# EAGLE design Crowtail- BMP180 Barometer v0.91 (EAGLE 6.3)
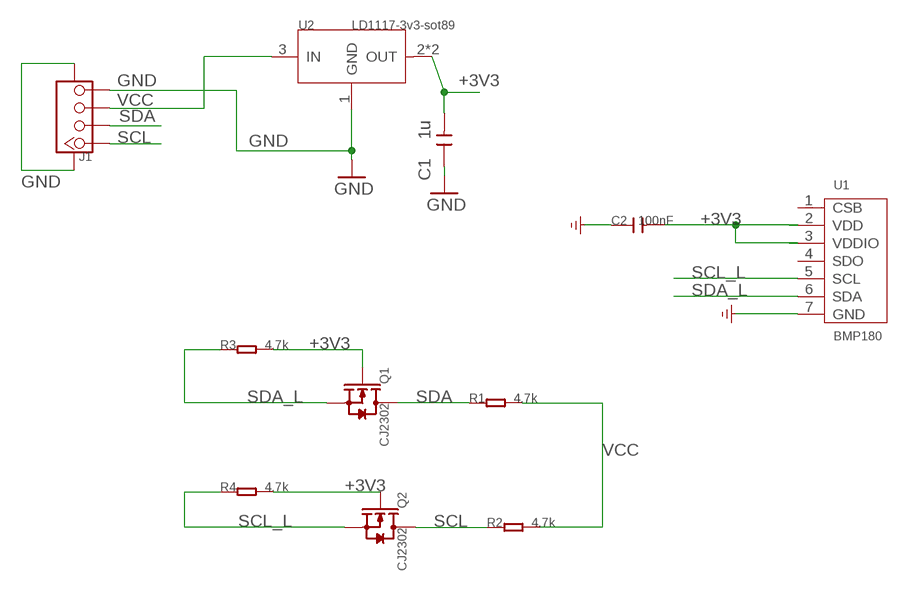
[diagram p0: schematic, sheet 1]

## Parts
C1  1u  C-0603  [C0603]
C2  100nF  C-0603  [C0603]
J1  TWIG-4P-2.0-SMD-FEMALE-REINFORCE'90D'  [4P-SMD-2.0-90D]
Q1  CJ2302  MOSFET-N-044020001  [SOT23]
Q2  CJ2302  MOSFET-N-044020001  [SOT23]
R1  4.7k  R-0603  [R0603]
R2  4.7k  R-0603  [R0603]
R3  4.7k  R-0603  [R0603]
R4  4.7k  R-0603  [R0603]
U1  BMP180  [LGA-7]
U2  LD1117-3v3-sot89  LD1117'SOT89'  [SOT89]

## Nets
+3V3 [power]: C1.2 C2.2 Q1.1(G) Q2.1(G) R3.2 R4.2 U1.2(VDD) U1.3(VDDIO) U2.2(OUT) U2.4(OUT)
GND: C1.1 C2.1 J1.4 J1.SS1 J1.SS2 U1.7(GND) U2.1(GND)
SCL: J1.1 Q2.3(D) R2.1
SCL_L: Q2.2(S) R4.1 U1.5(SCL)
SDA: J1.2 Q1.3(D) R1.1
SDA_L: Q1.2(S) R3.1 U1.6(SDA)
VCC: J1.3 R1.2 R2.2 U2.3(IN)
Unconnected: U1.1(CSB) U1.4(SDO)

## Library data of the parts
C1 C2 = Discrete:C*: Ceramic Capacitors
J1 = Connector:TWIG-4P-2.0-SMD-FEMALE-REINFORCE
Q1 Q2 = OPL:MOSFET-N: CJ2302：SMD MOSFET N-CH 20V-2.1A
R1-R4 = Discrete:R*
U1 = template :BMP180: Digital pressure sensor
U2 = IC:LD1117: Low Drop Fixed And Adjustable Positive Voltage Regulators http://www.datasheetcatalog.org/datasheet/SGSThomsonMicroelectronics/mXuqtqv.pdf

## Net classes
1 power: width 0.61 mm, drill 0.406 mm, clearance 0.203 mm
2 gnd: width 0.305 mm, drill 0.559 mm, clearance 0.254 mm
3 usbvcc: width 0.508 mm, drill 0.61 mm, clearance 0.254 mm

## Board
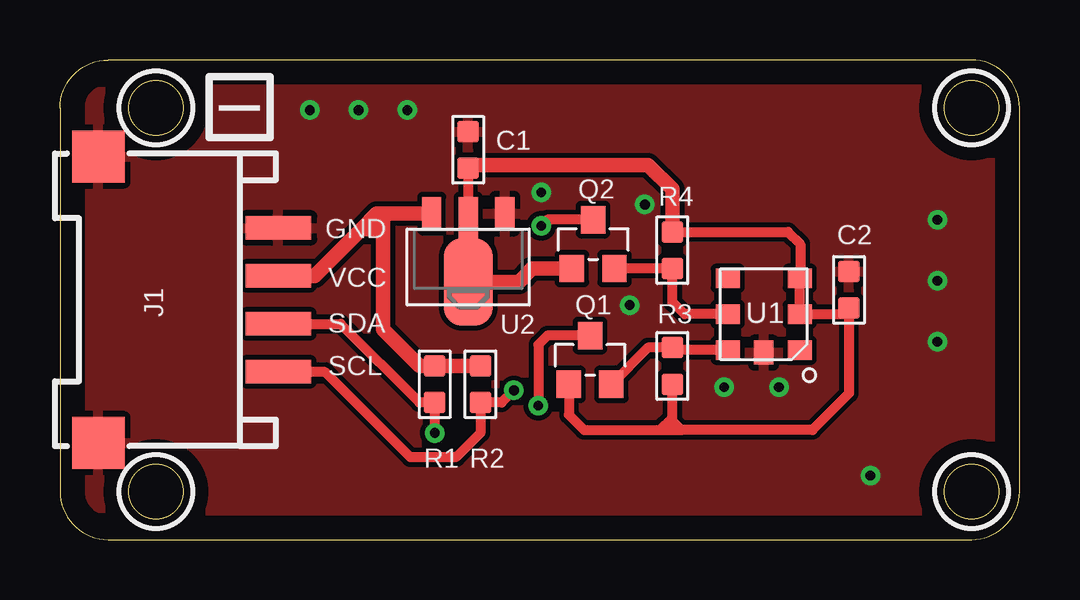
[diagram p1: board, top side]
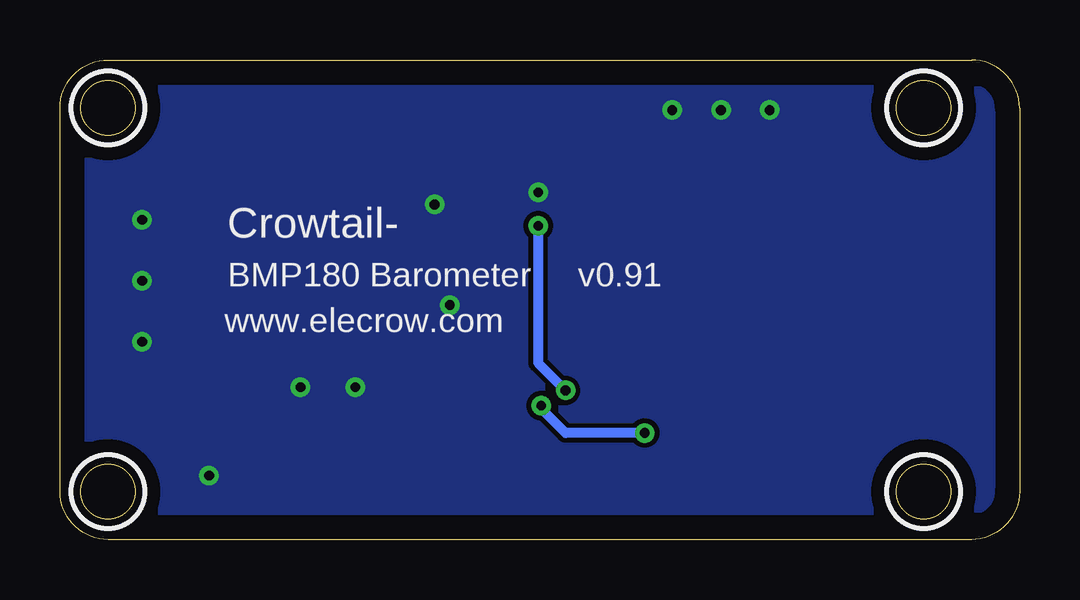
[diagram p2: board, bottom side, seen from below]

Size 40 x 20 mm. Coordinates in mm from the lower left corner, seen from the top.
Outline: 0,18 0,2 arc90 2,0 38,0 arc90 40,2 40,18 arc90 38,20 2,20 arc90 0,18
Outline: circle at 4,18 radius 1.14
Outline: circle at 4,2 radius 1.14
Outline: circle at 38,18 radius 1.14
Outline: circle at 38,2 radius 1.14
Copper layers (1*16): Top 0.035mm / dielectric 1.5mm / Bottom 0.035mm
Design rules "default *": minimum track width 10mil, minimum drill 24mil, track to track 8mil, track to pad 8mil, pad to pad 8mil, via to via 8mil, smd to smd 8mil, copper to edge 40mil, drill to drill 8mil, minimum pad ring 10mil, minimum via ring 8mil, stop-mask expansion 2mil, vias tented up to drill 100mil, thermal gap 10mil
tRestrict: area 2.5,16.5 to 5.5,19.5; area 2.5,0.5 to 5.5,3.5; area 36.5,16.5 to 39.5,19.5; area 36.5,0.5 to 39.5,3.5
bRestrict: area 2.5,16.5 to 5.5,19.5; area 2.5,0.5 to 5.5,3.5; area 36.5,16.5 to 39.5,19.5; area 36.5,0.5 to 39.5,3.5

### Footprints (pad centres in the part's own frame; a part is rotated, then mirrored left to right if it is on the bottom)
C0603 = smd 0.889 x 0.889: 1 -0.762,0; 2 0.762,0
4P-SMD-2.0-90D = smd 0.965 x 2.74: 1 -3,-0.1; 2 -1,-0.1; 3 1,-0.1; 4 3,-0.1 | smd 2.159 x 2.184: SS1 -5.974,7.4; SS2 5.974,7.4
SOT23 = smd 1.016 x 1.143: 1 -0.889,-1.016; 2 0.889,-1.016; 3 0,1.016
R0603 = smd 0.889 x 0.889: 1 -0.762,0; 2 0.762,0
LGA-7 = smd 0.8 x 1: 1 1.5,1.5; 2 0,1.5; 3 -1.5,1.5; 4 -1.5,-1.5; 5 0,-1.5; 6 1.5,-1.5 | smd 1 x 0.8: 7 1.6,0
SOT89 = smd 0.8 x 1.4: 1 -1.524,-1.905; 3 1.524,-1.905 | smd 0.8 x 1.9: 2 0,-1.651 | smd 2.032 x 3.65: 4 0,0.94

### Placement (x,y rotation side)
C1  17.02,16.26 270 top
C2  32.89,10.41 270 top
J1  9,10 90 top
Q1  22.1,7.49 0 top
Q2  22.23,12.32 0 top
R1  15.62,6.48 90 top
R2  17.53,6.48 90 top
R3  25.53,7.24 270 top
R4  25.53,12.06 90 top
U1  29.34,9.4 270 top
U2  17.02,11.68 180 top

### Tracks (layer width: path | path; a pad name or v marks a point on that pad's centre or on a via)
+3V3
  Top 0.406: C1.2 U2.2 U2.4 | Q1.1 21.21,5.21 21.84,4.57 25.02,4.57 | 25.02,4.57 25.91,4.57 | 25.53,5.08 25.53,4.95 25.91,4.57 | 25.53,5.08 R3.2 | R4.2 30.35,12.83 30.86,12.32 30.86,10.92 U1.3 U1.2 32.64,9.4 C2.2 32.89,6.1 31.37,4.57 25.91,4.57 | 25.02,4.57 25.53,5.08
  Top 0.61: U2.4 19.13,10.74 19.68,11.3 Q2.1 | R4.2 25.53,14.61 24.51,15.62 17.14,15.62 C1.2
GND  (via drill 0.41)
  other vias: 36.58,13.34 36.58,10.79 36.58,8.26 27.69,6.35 24.38,13.97 10.41,17.91 12.45,17.91 14.48,17.91 20.07,14.48 29.97,6.35 33.78,2.67 23.75,9.78
  pour Top: 0,20.32 40.64,20.32 40.64,0 0,0
  pour Bottom: 0,20.32 40.64,20.32 40.64,0 0,0
SCL  (via drill 0.41)
  Top 0.406: Q2.3 20.32,13.34 v20.07,13.08 | J1.1 9.12,6.99 11.05,6.99 14.61,3.43 16.51,3.43 17.53,4.45 R2.1 18.41,5.71 v18.92,6.22
  Bottom 0.406: v20.07,13.08 20.07,7.37 v18.92,6.22
SCL_L
  Top 0.406: U1.5 26.04,9.4 25.53,9.91 R4.1 Q2.2
SDA  (via drill 0.41)
  Top 0.406: Q1.3 20.32,8.51 19.94,8.13 v19.94,5.59 | J1.2 11.7,9 14.99,5.71 R1.1 v15.62,4.45
  Bottom 0.406: v19.94,5.59 19.94,5.46 18.92,4.45 v15.62,4.45
SDA_L
  Top 0.406: U1.6 25.63,7.9 R3.1 24.51,8 Q1.2
VCC
  Top 0.61: J1.3 10.62,11 12.57,12.95 | 12.57,12.95 13.21,13.59 13.46,13.59 | 13.46,13.59 U2.3 | R2.2 R1.2 14.99,7.24 13.46,8.76 13.46,12.95 | 13.46,12.95 13.46,13.59 | 12.57,12.95 13.46,12.95

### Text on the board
tPlace: I | GND | VCC | SDA | SCL
bPlace: Crowtail- | v0.91 | BMP180 Barometer | www.elecrow.com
